|   IBIS model for TI xxx DSP
[IBIS Ver]   5.1
[Disclaimer]   Please be aware that in the absence of a written agreement
|   Texas Instruments(TI) assumes no liability for:
|   (1) The accuracy of the IBIS models provided to your company,
|   however, the IBIS model is compliant to industry standard
|   IQ Level 2a.  Refer to IBIS Quality Section below for
|   for full details.
|   (2) The proper functioning of these Models in your design
|   or for any resulting applications
|   (3) Infringement of patents, copyrights or intellectual
|   property rights resulting from your use of these
|   models.
|   TI provides IBIS Models as a service to our customers and
|   therefore reserves the right to limit distribution of the
|   Models.  The information is subject to change without notice.
[File Name]  dlp8430_v2.ibs
[File Rev]   0.2
|   -Initial version
|   -updated LVCMOS models
[Date]   11Sept2024
[Source]   Texas Instruments Incorporated
[Copyright]   Property of Texas Instruments Incorporated.
|   Unauthorized reproduction and/or distribution is strictly.
|   prohibited.
|   This product is protected under copyright law and trade
|   secret law as an unpublished work.
|   Created 2012,(C) Copyright 1999-2012,
|   Texas Instruments Incorporated., All Rights Reserved.
|   These commodities are under the U.S. Government
|   distribution license control. As such,they are not to be
|   re-exported without the prior approval of the U.S.
|   Department of Commerce.
[Notes]
   This file does not include AMI models for SerDes based links.
   For SerDes simulations use Texas Instruments IBIS AMI models
   Some IV curves contain Non monotonic data points.
|   Revision History
|   GERNERAL COMMENT: All IBIS Quality Notes below reflect latest release
|   and version of IBIS File
|   File passes ibischk6.0 with 0 errors and 139 warnings
|   Component DLP84xx
[Component] DLP84xx
[Manufacturer] Texas Instruments
[Package]
|Variable   Typ   Min   Max
R_pkg   0.139   0.031	0.325
L_pkg   1.052e-9   0.293e-9	2.336e-9
C_pkg   0.364e-12   0.208e-12	0.669e-12
[Package Model]   dlpc84xx_pkg
[Pin]  Signal_name   model_name
A1	VSS   GND
A3	DMD_HS0_WDATA0_P	LVDS
A5	DMD_HS0_WDATA3_P	LVDS
A7	DMD_HS0_WDATA5_P	LVDS
A9	VSS   GND
A11	DMD_HS1_WDATA1_P	LVDS
A13	DMD_HS1_CLK_P   LVDS
A15	DMD_HS1_WDATA6_P	LVDS
A17	DMD_HS2_WDATA0_P	LVDS
A19	DMD_HS2_CLK_P   LVDS
A21	DMD_HS2_WDATA5_P	LVDS
A23	VSS   GND
A25	VSS   GND
B2	DMD_LS0_WDATA_P   LVDS
B4	DMD_HS0_WDATA2_P	LVDS
B6	DMD_HS0_CLK_P   LVDS
B8	DMD_HS0_WDATA7_P	LVDS
B10	DMD_HS1_WDATA0_P	LVDS
B12	DMD_HS1_WDATA3_P	LVDS
B14	DMD_HS1_WDATA4_P	LVDS
B16	VSS   GND
B18	DMD_HS2_WDATA2_P	LVDS
B20	DMD_HS2_WDATA4_P	LVDS
B22	DMD_HS2_WDATA7_P	LVDS
B24	DMD_HS3_WDATA0_P	LVDS
C1	DMD_LS0_WDATA_N	LVDS
C3	DMD_HS0_WDATA0_N	LVDS
C5	DMD_HS0_WDATA3_N	LVDS
C7	DMD_HS0_WDATA5_N	LVDS
C9	VSS   GND
C11	DMD_HS1_WDATA1_N	LVDS
C13	DMD_HS1_CLK_N   LVDS
C15	DMD_HS1_WDATA6_N	LVDS
C17	DMD_HS2_WDATA0_N	LVDS
C19	DMD_HS2_CLK_N   LVDS
C21	DMD_HS2_WDATA5_N	LVDS
C23	VSS   GND
C25	DMD_HS3_WDATA0_N	LVDS
D2	VSS   GND
D4	DMD_HS0_WDATA2_N	LVDS
D6	DMD_HS0_CLK_N   LVDS
D8	DMD_HS0_WDATA7_N	LVDS
D10	DMD_HS1_WDATA0_N	LVDS
D12	DMD_HS1_WDATA3_N	LVDS
D14	DMD_HS1_WDATA4_N	LVDS
D16	VSS   GND
D18	DMD_HS2_WDATA2_N	LVDS
D20	DMD_HS2_WDATA4_N	LVDS
D22	DMD_HS2_WDATA7_N	LVDS
D24	DMD_HS3_WDATA1_P	LVDS
E1	DMD_LS0_CLK_N   LVDS
E3	DMD_LS1_WDATA   LVCMOS18_H
E5	DMD_HS0_WDATA1_N	LVDS
E7	DMD_HS0_WDATA4_N	LVDS
E9	DMD_HS0_WDATA6_N	LVDS
E11	DMD_HS1_WDATA2_N	LVDS
E13	DMD_HS1_WDATA5_N	LVDS
E15	DMD_HS1_WDATA7_N	LVDS
E17	DMD_HS2_WDATA1_N	LVDS
E19	DMD_HS2_WDATA3_N	LVDS
E21	DMD_HS2_WDATA6_N	LVDS
E23	DMD_HS3_WDATA2_N	LVDS
E25	DMD_HS3_WDATA1_N	LVDS
F2	DMD_LS0_CLK_P   LVDS
F4	DMD_HS0_WDATA1_P	LVDS
F6	DMD_HS0_WDATA4_P	LVDS
F8	DMD_HS0_WDATA6_P	LVDS
F10	DMD_HS1_WDATA2_P	LVDS
F12	DMD_HS1_WDATA5_P	LVDS
F14	DMD_HS1_WDATA7_P	LVDS
F16	DMD_HS2_WDATA1_P	LVDS
F18	DMD_HS2_WDATA3_P	LVDS
F20	DMD_HS2_WDATA6_P	LVDS
F22	DMD_HS3_WDATA2_P	LVDS
F24	DMD_HS3_WDATA3_P	LVDS
G1	DMD_LS1_CLK   LVCMOS18_H
G3	DMD_LS2_WDATA   LVCMOS18_H
G5	VSS   GND
G7	VSS   GND
G9	VSS   GND
G11	VSS   GND
G13	ATEST   NC
G15	VSS   GND
G17	VSS   GND
G19	VSS   GND
G21	VSS   GND
G23	DMD_HS3_WDATA4_N	LVDS
G25	DMD_HS3_WDATA3_N	LVDS
H2	DMD_LS2_CLK   LVCMOS18_H
H4	DMD_LS0_RDATA   LVCMOS18_H
H6	VSS   GND
H8	VSS   GND
H10	VSS   GND
H12	VSS   GND
H14	VSS   GND
H16	VSS   GND
H18	VSS   GND
H20	VSS   GND
H22	DMD_HS3_WDATA4_P	LVDS
H24	DMD_HS3_CLK_P   LVDS
J1	DMD_DEN_ARSTZ   LVCMOS18_H
J3	DMD_LS1_RDATA   LVCMOS18_H
J5	VSS   GND
J7	VDDA18_DDI   POWER
J9	VDDA18_DDI   POWER
J11	VDDA18_DDI   POWER
J13	VDDA18_PLLD   POWER
J15	VDDA18_DDI   POWER
J17	VDDA18_DDI   POWER
J19	VDDA18_DDI   POWER
J21	VSS   GND
J23	DMD_HS3_WDATA6_N	LVDS
J25	DMD_HS3_CLK_N   LVDS
K2	VSENSE   NC
K4	DMD_LS3_RDATA   LVCMOS18_H
K6	VSS   GND
K8	VDD_CORE   POWER
K10	VSS   GND
K16	VSS   GND
K18	VDD_CORE   POWER
K20	VSS   GND
K22	DMD_HS3_WDATA6_P	LVDS
K24	DMD_HS3_WDATA5_P	LVDS
L1	PLL_REFCLK_O   NC
L3	IFORCE   NC
L5	VSS   GND
L7	VSS   GND
L9	VDD_CORE   POWER
L11	VSS   GND
L13	VDD_CORE   POWER
L15	VSS   GND
L17	VSS   GND
L21	VPP   NC
L23	DMD_HS3_WDATA7_N	LVDS
L25	DMD_HS3_WDATA5_N	LVDS
M2	VSS   GND
M4	DMD_LS2_RDATA   LVCMOS18_H
M6	VDD_CORE   POWER
M10	VSS   GND
M14	VSS   GND
M18	VSS   GND
M20	VDD_CORE   POWER
M22	DMD_HS3_WDATA7_P	LVDS
M24	TSTPT_7   LVCMOS18_H
N1	PLL_REFCLK_I   NC
N3	GPIO_09   LVCMOS18_H
N5	VSS   GND
N7	VSS   GND
N11	VDDAR_CORE   POWER
N13	VDDAR_CORE   POWER
N15	VDD_CORE   POWER
N17	VDD_CORE   POWER
N21	VDDS18_LVCMOS2   POWER
N23	TSTPT_6   LVCMOS18_H
N25	TSTPT_4   LVCMOS18_H
P2	RESETZ   RESET_H
P4	GPIO_10   LVCMOS18_H
P8	VDDAR_CORE   POWER
P10	VSS   GND
P12	VSS   GND
P14	VSS   GND
P18	VDDAR_CORE   POWER
P20	VSS   GND
P22	TSTPT_5   LVCMOS18_H
P24	TSTPT_3   LVCMOS18_H
R1	GPIO_19   LVCMOS18_H
R3	GPIO_20   LVCMOS18_H
R5	VSS   GND
R9	VDDAR_CORE   POWER
R11	VSS   GND
R15	VSS   GND
R17	VSS   GND
R19	VDDAR_CORE   POWER
R21	VDDS18_LVCMOS2   POWER
R23	TSTPT_2   LVCMOS18_H
R25	TSTPT_1   LVCMOS18_H
T2	GPIO_22   LVCMOS18_H
T4	GPIO_11   LVCMOS18_H
T6	VDD_CORE   POWER
T8	VSS   GND
T10	VSS   GND
T12	VDD_CORE   POWER
T14	VDD_CORE   POWER
T16	VSS   GND
T20	VDD_CORE   POWER
T22	TSTPT_0   LVCMOS18_H
T24	ETM_TRACECTL   LVCMOS18_H
U1	GPIO_21   LVCMOS18_H
U3	GPIO_23   LVCMOS18_H
U5	VDDS18_OSC   POWER
U7	VSS   GND
U11	VSS   GND
U15	VSS   GND
U17	VSS   GND
U19	VDD_CORE   POWER
U21	VDDS18_LVCMOS2   POWER
U23	JTAGTMS1   LVCMOS18_H
U25	ETM_TRACECLK   LVCMOS18_H
V2	GPIO_25   LVCMOS18_H
V4	GPIO_12   LVCMOS18_H
V6	VSS   GND
V8	VDD_CORE   POWER
V10	VDD_CORE   POWER
V12	VSS   GND
V14	VSS   GND
V20	VSS   GND
V22	JTAGTDO1   LVCMOS18_H
V24	JTAGTCK   LVCMOS18_H
W1	GPIO_24   LVCMOS18_H
W3	GPIO_26   LVCMOS18_H
W5	VDDS18_LVCMOS1   POWER
W7	VSS   GND
W13	VSS   GND
W15	VDDAR_CORE   POWER
W17	VDDAR_CORE   POWER
W19	VSS   GND
W21	VDDS18_LVCMOS2   POWER
W23	JTAGTDO2   LVCMOS18_H
W25	JTAGTMS2   LVCMOS18_H
Y2	GPIO_29   LVCMOS18_H
Y4	GPIO_28   LVCMOS18_H
Y6	VDD_CORE   POWER
Y8	VSS   GND
Y10	VSS   GND
Y12	VSS   GND
Y14	VSS   GND
Y18	VSS   GND
Y20	VDD_CORE   POWER
Y22	HWTEST_EN   LVCMOS18_H
Y24	JTAGTDI   LVCMOS18_H
AA1	GPIO_27   LVCMOS18_H
AA3	GPIO_30   LVCMOS18_H
AA5	VDDS18_LVCMOS1   POWER
AA7	VSS   GND
AA9	VSS   GND
AA13	VDD_CORE   POWER
AA15	VDD_CORE   POWER
AA17	VSS   GND
AA19	VSS   GND
AA21	VDD_CORE   POWER
AA23	GPTP0   LVCMOS18_H
AA25	JTAGTRSTZ   LVCMOS18_H
AB2	GPIO_33   LVCMOS18_H
AB4	GPIO_31   LVCMOS18_H
AB6	VSS   GND
AB8	VSS   GND
AB10	VDDAR_CORE   POWER
AB12	VDDAR_CORE   POWER
AB14	VSS   GND
AB16	VDD_CORE   POWER
AB18	VSS   GND
AB20	VSS   GND
AB22	GPTP1   LVCMOS18_H
AB24	OCLKA   LVCMOS18_H
AC1	GPIO_32   LVCMOS18_H
AC3	GPIO_34   LVCMOS18_H
AC5	VSS   GND
AC9	VSS   GND
AC11	VSS   GND
AC13	VDD_CORE   POWER
AC15	VSS   GND
AC17	VSS   GND
AC21	VDDSHV_FLSH   POWER
AC23	GPIO_14   LVCMOS18_H
AC25	GPTP2   LVCMOS18_H
AD2	GPIO_37   LVCMOS18_H
AD4	GPIO_35   LVCMOS18_H
AD6	VDD_CORE   POWER
AD8	VDD_CORE   POWER
AD12	VSS   GND
AD14	VSS   GND
AD16	VSS   GND
AD18	VDD_CORE   POWER
AD20	VDD_CORE   POWER
AD22	CAP_VDDS_FLSH   POWER
AD24	GPIO_13   LVCMOS18_H
AE1	GPIO_36   LVCMOS18_H
AE3	GPIO_38   LVCMOS18_H
AE5	VDDS18_LVCMOS1   POWER
AE9	VDD_CORE   POWER
AE11	VDD_CORE   POWER
AE13	VSS   GND
AE17	VSS   GND
AE21	VDDSHV_FLSH   POWER
AE23	GPIO_16   LVCMOS18_H
AE25	GPIO_15   LVCMOS18_H
AF2	GPIO_41   LVCMOS18_H
AF4	GPIO_40   LVCMOS18_H
AF6	VSS   GND
AF8	VSS   GND
AF12	VSS   GND
AF14	VDD_CORE   POWER
AF16	VDD_CORE   POWER
AF18	VSS   GND
AF20	VDD_CORE   POWER
AF22	GPIO_18   LVCMOS18_H
AF24	GPIO_17   LVCMOS18_H
AG1	GPIO_39   LVCMOS18_H
AG3	GPIO_43   LVCMOS18_H
AG5	VDDS18_LVCMOS1   POWER
AG7	VDD_CORE   POWER
AG9	VSS   GND
AG11	VSS   GND
AG13	VSS   GND
AG17	VSS   GND
AG19	VSS   GND
AG21	VDDSHV_INTF   POWER
AG23	FLSH_CSZ   SDIO_H
AG25	FLSH_CLK   SDIO_H
AH2	GPIO_44   LVCMOS18_H
AH4	ATB_0_H   NC
AH6	VDD_CORE   POWER
AH10	VSS   GND
AH14	VSS   GND
AH16	VSS   GND
AH20	VSS   GND
AH22	FLSH_DATA0   SDIO_H
AH24	FLSH_DATA1   SDIO_H
AJ1	GPIO_42   LVCMOS18_H
AJ3	GPIO_45   LVCMOS18_H
AJ5	ATB_1_H   NC
AJ9	VDDAR_CORE   POWER
AJ11	VDD_CORE   POWER
AJ13	VDDAR_CORE   POWER
AJ15	VDDAR_CORE   POWER
AJ17	VDDAR_CORE   POWER
AJ19	VDDAR_CORE   POWER
AJ21	CAP_VDDS_INTF   POWER
AJ23	FLSH_DATA3   SDIO_H
AJ25	FLSH_DATA2   SDIO_H
AK2	GPIO_48   LVCMOS18_H
AK4	GPIO_47   LVCMOS18_H
AK6	VSS   GND
AK8	VDDAR_CORE   POWER
AK16	VSS   GND
AK20	VSS   GND
AK22	HOST_IRQ   LVCMOS1833_H
AK24	IIC0_SDA   IIC_H
AL1	GPIO_46   LVCMOS18_H
AL3	GPIO_50   LVCMOS18_H
AL5	VDDS18_LVCMOS1   POWER
AL7	VSS   GND
AL9	VDD_CORE   POWER
AL11	VDDA18_PLLM   POWER
AL13	VDD_CORE   POWER
AL15	VSS   GND
AL17	VDD_CORE   POWER
AL19	VDD_CORE   POWER
AL21	VDDSHV_INTF   POWER
AL23	GPIO_07   LVCMOS1833_H
AL25	IIC0_SCL   IIC_H
AM2	GPIO_51   LVCMOS18_H
AM4	P1_LOCKN   LVCMOS18_H
AM6	VDDA_CORE_USB   POWER
AM8	VSS   GND
AM10	VDDA_CORE_VX1   POWER
AM12	VDDA18_VX1   POWER
AM14	VDDA_CORE_VX1   POWER
AM16	VDDA_CORE_FPD   POWER
AM18	VDDA_CORE_FPD   POWER
AM20	VDDA_CORE_FPD   POWER
AM22	SSP0_CSZ_0   LVCMOS1833_H
AM24	GPIO_08   LVCMOS1833_H
AN1	GPIO_49   LVCMOS18_H
AN3	P1_HTPDN   LVCMOS18_H
AN5	VSS   GND
AN7	VDDA18_USB   POWER
AN9	VSS   GND
AN15	VDDA18_FPD   POWER
AN21	VSS   GND
AN23	SSP0_DI   LVCMOS1833_H
AN25	SSP0_CLK   LVCMOS1833_H
AP2	PROJ_ON   LVCMOS18_H
AP4	USB_VBUS   NC
AP6	VDDA33_USB   POWER
AP8	VDDA18_DSI   POWER
AP10	VDDA18_VX1   POWER
AP12	VSS   GND
AP14	VDDA18_VX1   POWER
AP16	VDDA18_FPD   POWER
AP18	VDDA18_FPD   POWER
AP20	VSS   GND
AP22	GPIO_06   LVCMOS1833_H
AP24	SSP0_DO   LVCMOS1833_H
AR1	PARKZ   LVCMOS18_H
AR3	USB_TXRTUNE   NC
AR5	VSS   GND
AR7	VDDA_CORE_DSI   POWER
AR9	VSS   GND
AR11	VSS   GND
AR13	VSS   GND
AR15	VSS   GND
AR17	VSS   GND
AR19	VDDA18_FPD   POWER
AR21	VSS   GND
AR23	GPIO_05   LVCMOS1833_H
AR25	GPIO_00   LVCMOS1833_H
AT2	USB_ID   NC
AT4	VSS   GND
AT6	VSS   GND
AT8	VSS   GND
AT10	VSS   GND
AT12	VSS   GND
AT14	VSS   GND
AT16	P2A_LVDS_RPI   NC
AT18	VSS   GND
AT20	P2B_LVDS_RPI   NC
AT22	VSS   GND
AT24	GPIO_03   LVCMOS1833_H
AU1	USB_DAT_P   NC
AU3	VSS   GND
AU5	P3_DSI_D2_N   NC
AU7	VSS   GND
AU9	P1_VX1_D0_N   VBO
AU11	P1_RREF   NC
AU13	P1_VX1_D5_N   VBO
AU15	P2A_LVDS_D2_N   FPD
AU17	P2A_LVDS_D4_N   FPD
AU19	P2B_LVDS_D1_N   FPD
AU21	P2B_LVDS_D2_N   FPD
AU23	VSS   GND
AU25	GPIO_01   LVCMOS1833_H
AV2	VSS   GND
AV4	P3_DSI_D2_P   NC
AV6	P3_DSI_RCALIB   NC
AV8	P1_VX1_D0_P   VBO
AV10	VSS   GND
AV12	P1_VX1_D5_P   NC
AV14	VSS   GND
AV16	P2A_LVDS_D2_P   FPD
AV18	P2A_LVDS_D4_P   FPD
AV20	P2B_LVDS_D1_P   FPD
AV22	P2B_LVDS_D2_P   FPD
AV24	GPIO_04   LVCMOS1833_H
AW1	USB_DAT_N   NC
AW3	P3_DSI_D3_N   NC
AW5	P3_DSI_D0_N   NC
AW7	VSS   GND
AW9	P1_VX1_D2_N   VBO
AW11	P1_VX1_D4_N   VBO
AW13	P1_VX1_D7_N   VBO
AW15	P2A_LVDS_D0_N   FPD
AW17	P2A_LVDS_C_N   FPD
AW19	VSS   GND
AW21	P2B_LVDS_C_N   FPD
AW23	P2B_LVDS_D4_N   FPD
AW25	GPIO_02   LVCMOS1833_H
AY2	VSS   GND
AY4	P3_DSI_D1_N   NC
AY6	P3_DSI_C_N   NC
AY8	P1_VX1_D1_N   VBO
AY10	P1_VX1_D3_N   VBO
AY12	P1_VX1_D6_N   VBO
AY14	VSS   GND
AY16	P2A_LVDS_D1_N   FPD
AY18	P2A_LVDS_D3_N   FPD
AY20	P2B_LVDS_D0_N   FPD
AY22	P2B_LVDS_D3_N   FPD
AY24	VSS   GND
BA1	VSS   GND
BA3	P3_DSI_D3_P   NC
BA5	P3_DSI_D0_P   NC
BA7	VSS   GND
BA9	P1_VX1_D2_P   VBO
BA11	P1_VX1_D4_P   VBO
BA13	P1_VX1_D7_P   VBO
BA15	P2A_LVDS_D0_P   FPD
BA17	P2A_LVDS_C_P   FPD
BA19	VSS   GND
BA21	P2B_LVDS_C_P   FPD
BA23	P2B_LVDS_D4_P   FPD
BA25	VSS   GND
BB2	VSS   GND
BB4	P3_DSI_D1_P   NC
BB6	P3_DSI_C_P   NC
BB8	P1_VX1_D1_P   VBO
BB10	P1_VX1_D3_P   VBO
BB12	P1_VX1_D6_P   VBO
BB14	VSS   GND
BB16	P2A_LVDS_D1_P   FPD
BB18	P2A_LVDS_D3_P   FPD
BB20	P2B_LVDS_D0_P   FPD
BB22	P2B_LVDS_D3_P   FPD
BB24	VSS   GND
|********************  DIFF PIN  *******************************
[Diff_pin]   inv_pin vdiff tdelay_typ   tdelay_min  tdelay_max
B6   D6   NA NA NA NA	||	DMD_HS0_CLK_P && DMD_HS0_CLK_N
A3   C3   NA NA NA NA	||	DMD_HS0_WDATA0_P && DMD_HS0_WDATA0_N
F4   E5   NA NA NA NA	||	DMD_HS0_WDATA1_P && DMD_HS0_WDATA1_N
B4   D4   NA NA NA NA	||	DMD_HS0_WDATA2_P && DMD_HS0_WDATA2_N
A5   C5   NA NA NA NA	||	DMD_HS0_WDATA3_P && DMD_HS0_WDATA3_N
F6   E7   NA NA NA NA	||	DMD_HS0_WDATA4_P && DMD_HS0_WDATA4_N
A7   C7   NA NA NA NA	||	DMD_HS0_WDATA5_P && DMD_HS0_WDATA5_N
F8   E9   NA NA NA NA	||	DMD_HS0_WDATA6_P && DMD_HS0_WDATA6_N
B8   D8   NA NA NA NA	||	DMD_HS0_WDATA7_P && DMD_HS0_WDATA7_N
A13   C13   NA NA NA NA	||	DMD_HS1_CLK_P && DMD_HS1_CLK_N
B10   D10   NA NA NA NA	||	DMD_HS1_WDATA0_P && DMD_HS1_WDATA0_N
A11   C11   NA NA NA NA	||	DMD_HS1_WDATA1_P && DMD_HS1_WDATA1_N
F10   E11   NA NA NA NA	||	DMD_HS1_WDATA2_P && DMD_HS1_WDATA2_N
B12   D12   NA NA NA NA	||	DMD_HS1_WDATA3_P && DMD_HS1_WDATA3_N
B14   D14   NA NA NA NA	||	DMD_HS1_WDATA4_P && DMD_HS1_WDATA4_N
F12   E13   NA NA NA NA	||	DMD_HS1_WDATA5_P && DMD_HS1_WDATA5_N
A15   C15   NA NA NA NA	||	DMD_HS1_WDATA6_P && DMD_HS1_WDATA6_N
F14   E15   NA NA NA NA	||	DMD_HS1_WDATA7_P && DMD_HS1_WDATA7_N
A19   C19   NA NA NA NA	||	DMD_HS2_CLK_P && DMD_HS2_CLK_N
A17   C17   NA NA NA NA	||	DMD_HS2_WDATA0_P && DMD_HS2_WDATA0_N
F16   E17   NA NA NA NA	||	DMD_HS2_WDATA1_P && DMD_HS2_WDATA1_N
B18   D18   NA NA NA NA	||	DMD_HS2_WDATA2_P && DMD_HS2_WDATA2_N
F18   E19   NA NA NA NA	||	DMD_HS2_WDATA3_P && DMD_HS2_WDATA3_N
B20   D20   NA NA NA NA	||	DMD_HS2_WDATA4_P && DMD_HS2_WDATA4_N
A21   C21   NA NA NA NA	||	DMD_HS2_WDATA5_P && DMD_HS2_WDATA5_N
F20   E21   NA NA NA NA	||	DMD_HS2_WDATA6_P && DMD_HS2_WDATA6_N
B22   D22   NA NA NA NA	||	DMD_HS2_WDATA7_P && DMD_HS2_WDATA7_N
H24   J25   NA NA NA NA	||	DMD_HS3_CLK_P && DMD_HS3_CLK_N
B24   C25   NA NA NA NA	||	DMD_HS3_WDATA0_P && DMD_HS3_WDATA0_N
D24   E25   NA NA NA NA	||	DMD_HS3_WDATA1_P && DMD_HS3_WDATA1_N
F22   E23   NA NA NA NA	||	DMD_HS3_WDATA2_P && DMD_HS3_WDATA2_N
F24   G25   NA NA NA NA	||	DMD_HS3_WDATA3_P && DMD_HS3_WDATA3_N
H22   G23   NA NA NA NA	||	DMD_HS3_WDATA4_P && DMD_HS3_WDATA4_N
K24   L25   NA NA NA NA	||	DMD_HS3_WDATA5_P && DMD_HS3_WDATA5_N
K22   J23   NA NA NA NA	||	DMD_HS3_WDATA6_P && DMD_HS3_WDATA6_N
M22   L23   NA NA NA NA	||	DMD_HS3_WDATA7_P && DMD_HS3_WDATA7_N
F2   E1   NA NA NA NA	||	DMD_LS0_CLK_P && DMD_LS0_CLK_N
B2   C1   NA NA NA NA	||	DMD_LS0_WDATA_P && DMD_LS0_WDATA_N
AV8   AU9   NA NA NA NA	||	P1_VX1_D0_P && P1_VX1_D0_N
BB8   AY8   NA NA NA NA	||	P1_VX1_D1_P && P1_VX1_D1_N
BA9   AW9   NA NA NA NA	||	P1_VX1_D2_P && P1_VX1_D2_N
BB10   AY10   NA NA NA NA	||	P1_VX1_D3_P && P1_VX1_D3_N
BA11   AW11   NA NA NA NA	||	P1_VX1_D4_P && P1_VX1_D4_N
AV12   AU13   NA NA NA NA	||	P1_VX1_D5_P && P1_VX1_D5_N
BB12   AY12   NA NA NA NA	||	P1_VX1_D6_P && P1_VX1_D6_N
BA13   AW13   NA NA NA NA	||	P1_VX1_D7_P && P1_VX1_D7_N
BA17   AW17   NA NA NA NA	||	P2A_LVDS_C_P && P2A_LVDS_C_N
BA15   AW15   NA NA NA NA	||	P2A_LVDS_D0_P && P2A_LVDS_D0_N
BB16   AY16   NA NA NA NA	||	P2A_LVDS_D1_P && P2A_LVDS_D1_N
AV16   AU15   NA NA NA NA	||	P2A_LVDS_D2_P && P2A_LVDS_D2_N
BB18   AY18   NA NA NA NA	||	P2A_LVDS_D3_P && P2A_LVDS_D3_N
AV18   AU17   NA NA NA NA	||	P2A_LVDS_D4_P && P2A_LVDS_D4_N
BA21   AW21   NA NA NA NA	||	P2B_LVDS_C_P && P2B_LVDS_C_N
BB20   AY20   NA NA NA NA	||	P2B_LVDS_D0_P && P2B_LVDS_D0_N
AV20   AU19   NA NA NA NA	||	P2B_LVDS_D1_P && P2B_LVDS_D1_N
AV22   AU21   NA NA NA NA	||	P2B_LVDS_D2_P && P2B_LVDS_D2_N
BB22   AY22   NA NA NA NA	||	P2B_LVDS_D3_P && P2B_LVDS_D3_N
BA23   AW23   NA NA NA NA	||	P2B_LVDS_D4_P && P2B_LVDS_D4_N
|******************** LVDS ***********************************
[Model Selector] LVDS
lvds_tx_01   LVDS TX Driver Permumentation 01
lvds_tx_02   LVDS TX Driver Permumentation 02
lvds_tx_03   LVDS TX Driver Permumentation 03
lvds_tx_04   LVDS TX Driver Permumentation 04
lvds_tx_05   LVDS TX Driver Permumentation 05
lvds_tx_06   LVDS TX Driver Permumentation 06
lvds_tx_07   LVDS TX Driver Permumentation 07
lvds_tx_08   LVDS TX Driver Permumentation 08
lvds_tx_09   LVDS TX Driver Permumentation 09
lvds_tx_10   LVDS TX Driver Permumentation 10
lvds_tx_11   LVDS TX Driver Permumentation 11
lvds_tx_12   LVDS TX Driver Permumentation 12
lvds_tx_13   LVDS TX Driver Permumentation 13
lvds_tx_14   LVDS TX Driver Permumentation 14
lvds_tx_15   LVDS TX Driver Permumentation 15
lvds_tx_16   LVDS TX Driver Permumentation 16
lvds_tx_17   LVDS TX Driver Permumentation 17
lvds_tx_18   LVDS TX Driver Permumentation 18
lvds_tx_19   LVDS TX Driver Permumentation 19
lvds_tx_20   LVDS TX Driver Permumentation 20
lvds_tx_21   LVDS TX Driver Permumentation 21
lvds_tx_22   LVDS TX Driver Permumentation 22
lvds_tx_23   LVDS TX Driver Permumentation 23
lvds_tx_24   LVDS TX Driver Permumentation 24
|****************** SDIO **************************************
[Model Selector] SDIO_H
sdio1_r33_1p8_h PRWDWUWSWEWCDGSDIO_H@_R33_1p8_comment
sdio1_r33_3p3_h PRWDWUWSWEWCDGSDIO_H@_R33_3p3_comment
sdio1_r40_1p8_h PRWDWUWSWEWCDGSDIO_H@_R40_1p8_comment
sdio1_r40_3p3_h PRWDWUWSWEWCDGSDIO_H@_R40_3p3_comment
sdio1_r50_1p8_h PRWDWUWSWEWCDGSDIO_H@_R50_1p8_comment
sdio1_r50_3p3_h PRWDWUWSWEWCDGSDIO_H@_R50_3p3_comment
sdio1_r66_1p8_h PRWDWUWSWEWCDGSDIO_H@_R66_1p8_comment
sdio1_r66_3p3_h PRWDWUWSWEWCDGSDIO_H@_R66_3p3_comment
sdio1_utr33_1p8_h PRWDWUWSWEWCDGSDIO_H@_UT_R33_1p8_comment
sdio1_utr33_3p3_h PRWDWUWSWEWCDGSDIO_H@_UT_R33_3p3_comment
sdio1_utr40_1p8_h PRWDWUWSWEWCDGSDIO_H@_UT_R40_1p8_comment
sdio1_utr40_3p3_h PRWDWUWSWEWCDGSDIO_H@_UT_R40_3p3_comment
sdio1_utr50_1p8_h PRWDWUWSWEWCDGSDIO_H@_UT_R50_1p8_comment
sdio1_utr50_3p3_h PRWDWUWSWEWCDGSDIO_H@_UT_R50_3p3_comment
sdio1_utr66_1p8_h PRWDWUWSWEWCDGSDIO_H@_UT_R66_1p8_comment
sdio1_utr66_3p3_h PRWDWUWSWEWCDGSDIO_H@_UT_R66_3p3_comment
|********************I2C************************************
[Model Selector] IIC_V
IIC18_1_0_V PRBOPDDGZIIC_V@HSMODE_HSMCSE=0_0_comment 1.8V
IIC18_1_1_V PRBOPDDGZIIC_V@HSMODE_HSMCSE=0_1_comment 1.8V
IIC18_1_2_V PRBOPDDGZIIC_V@HSMODE_HSMCSE=1_0_comment 1.8V
IIC18_1_3_V PRBOPDDGZIIC_V@HSMODE_HSMCSE=1_1_comment 1.8V
IIC33_1_0_V PRBOPDDGZIIC_V@HSMODE_HSMCSE=0_0_comment
IIC33_1_1_V PRBOPDDGZIIC_V@HSMODE_HSMCSE=0_1_comment
IIC33_1_2_V PRBOPDDGZIIC_V@HSMODE_HSMCSE=1_0_comment
IIC33_1_3_V PRBOPDDGZIIC_V@HSMODE_HSMCSE=1_1_comment
[Model Selector] IIC_H
Cell18_0_0_H PRBOPDDGZIIC_H@HSMODE_HSMCSE=0_0_comment 1.8V
Cell18_0_1_H PRBOPDDGZIIC_H@HSMODE_HSMCSE=0_1_comment 1.8V
Cell18_0_2_H PRBOPDDGZIIC_H@HSMODE_HSMCSE=1_0_comment 1.8V
Cell18_0_3_H PRBOPDDGZIIC_H@HSMODE_HSMCSE=1_1_comment 1.8V
Cell33_0_0_H PRBOPDDGZIIC_H@HSMODE_HSMCSE=0_0_comment
Cell33_0_1_H PRBOPDDGZIIC_H@HSMODE_HSMCSE=0_1_comment
Cell33_0_2_H PRBOPDDGZIIC_H@HSMODE_HSMCSE=1_0_comment
Cell33_0_3_H PRBOPDDGZIIC_H@HSMODE_HSMCSE=1_1_comment
|***************** RESET *********************************************
[Model Selector] RESET_H
reset18_0_0 PDIDGZRESET_H
| **************** LVCMOS18 ******************************************
[Model Selector] LVCMOS18_H
|Cell1_0 PRWDWUWHWSWDGZ_H@DS0_DS1_DS2_DS3_SL_PE_PS_SPU=0_0_0_0_0_0_0_0_comment
|Cell1_1 PRWDWUWHWSWDGZ_H@DS0_DS1_DS2_DS3_SL_PE_PS_SPU=0_0_0_0_1_0_0_0_comment
|Cell1_2 PRWDWUWHWSWDGZ_H@DS0_DS1_DS2_DS3_SL_PE_PS_SPU=0_0_0_1_0_0_0_0_comment
|Cell1_3 PRWDWUWHWSWDGZ_H@DS0_DS1_DS2_DS3_SL_PE_PS_SPU=0_0_0_1_1_0_0_0_comment
|Cell1_4 PRWDWUWHWSWDGZ_H@DS0_DS1_DS2_DS3_SL_PE_PS_SPU=0_0_1_0_0_0_0_0_comment
|Cell1_5 PRWDWUWHWSWDGZ_H@DS0_DS1_DS2_DS3_SL_PE_PS_SPU=0_0_1_0_1_0_0_0_comment
|Cell1_6 PRWDWUWHWSWDGZ_H@DS0_DS1_DS2_DS3_SL_PE_PS_SPU=0_0_1_1_0_0_0_0_comment
|Cell1_7 PRWDWUWHWSWDGZ_H@DS0_DS1_DS2_DS3_SL_PE_PS_SPU=0_0_1_1_1_0_0_0_comment
|Cell1_8 PRWDWUWHWSWDGZ_H@DS0_DS1_DS2_DS3_SL_PE_PS_SPU=0_1_0_0_0_0_0_0_comment
|Cell1_9 PRWDWUWHWSWDGZ_H@DS0_DS1_DS2_DS3_SL_PE_PS_SPU=0_1_0_0_1_0_0_0_comment
|Cell1_10 PRWDWUWHWSWDGZ_H@DS0_DS1_DS2_DS3_SL_PE_PS_SPU=0_1_0_1_0_0_0_0_comment
|Cell1_11 PRWDWUWHWSWDGZ_H@DS0_DS1_DS2_DS3_SL_PE_PS_SPU=0_1_0_1_1_0_0_0_comment
|Cell1_12 PRWDWUWHWSWDGZ_H@DS0_DS1_DS2_DS3_SL_PE_PS_SPU=0_1_1_0_0_0_0_0_comment
|Cell1_13 PRWDWUWHWSWDGZ_H@DS0_DS1_DS2_DS3_SL_PE_PS_SPU=0_1_1_0_1_0_0_0_comment
|Cell1_14 PRWDWUWHWSWDGZ_H@DS0_DS1_DS2_DS3_SL_PE_PS_SPU=0_1_1_1_0_0_0_0_comment
|Cell1_15 PRWDWUWHWSWDGZ_H@DS0_DS1_DS2_DS3_SL_PE_PS_SPU=0_1_1_1_1_0_0_0_comment
|Cell1_16 PRWDWUWHWSWDGZ_H@DS0_DS1_DS2_DS3_SL_PE_PS_SPU=1_0_0_0_0_0_0_0_comment
|Cell1_17 PRWDWUWHWSWDGZ_H@DS0_DS1_DS2_DS3_SL_PE_PS_SPU=1_0_0_0_1_0_0_0_comment
|Cell1_18 PRWDWUWHWSWDGZ_H@DS0_DS1_DS2_DS3_SL_PE_PS_SPU=1_0_0_1_0_0_0_0_comment
|Cell1_19 PRWDWUWHWSWDGZ_H@DS0_DS1_DS2_DS3_SL_PE_PS_SPU=1_0_0_1_1_0_0_0_comment
Cell1_20 PRWDWUWHWSWDGZ_H@DS0_DS1_DS2_DS3_SL_PE_PS_SPU=1_0_1_0_0_0_0_0_comment
Cell1_21 PRWDWUWHWSWDGZ_H@DS0_DS1_DS2_DS3_SL_PE_PS_SPU=1_0_1_0_1_0_0_0_comment
|Cell1_22 PRWDWUWHWSWDGZ_H@DS0_DS1_DS2_DS3_SL_PE_PS_SPU=1_0_1_1_0_0_0_0_comment
|Cell1_23 PRWDWUWHWSWDGZ_H@DS0_DS1_DS2_DS3_SL_PE_PS_SPU=1_0_1_1_1_0_0_0_comment
|Cell1_24 PRWDWUWHWSWDGZ_H@DS0_DS1_DS2_DS3_SL_PE_PS_SPU=1_1_0_0_0_0_0_0_comment
|Cell1_25 PRWDWUWHWSWDGZ_H@DS0_DS1_DS2_DS3_SL_PE_PS_SPU=1_1_0_0_1_0_0_0_comment
|Cell1_26 PRWDWUWHWSWDGZ_H@DS0_DS1_DS2_DS3_SL_PE_PS_SPU=1_1_0_1_0_0_0_0_comment
|Cell1_27 PRWDWUWHWSWDGZ_H@DS0_DS1_DS2_DS3_SL_PE_PS_SPU=1_1_0_1_1_0_0_0_comment
|Cell1_28 PRWDWUWHWSWDGZ_H@DS0_DS1_DS2_DS3_SL_PE_PS_SPU=1_1_1_0_0_0_0_0_comment
|Cell1_29 PRWDWUWHWSWDGZ_H@DS0_DS1_DS2_DS3_SL_PE_PS_SPU=1_1_1_0_1_0_0_0_comment
|Cell1_30 PRWDWUWHWSWDGZ_H@DS0_DS1_DS2_DS3_SL_PE_PS_SPU=1_1_1_1_0_0_0_0_comment
|Cell1_31 PRWDWUWHWSWDGZ_H@DS0_DS1_DS2_DS3_SL_PE_PS_SPU=1_1_1_1_1_0_0_0_comment
[Model Selector] LVCMOS1833_H
lvcmos1_nom_1p8_h PRWDWUWSWEWCDGLVCMOS_V@DS3_DS2_DS1_DS0=1_1_0_0_comment
lvcmos1_nom_3p3_h PRWDWUWSWEWCDGLVCMOS_V@DS3_DS2_DS1_DS0=1_1_0_0_comment
|lvcmos1_nom_1p8_h PRWDWUWSWEWCDGLVCMOS_H@_Nom_1p8_comment
|lvcmos1_nom_3p3_h PRWDWUWSWEWCDGLVCMOS_H@_Nom_3p3_comment
|vcmos1_slow_1p8_h PRWDWUWSWEWCDGLVCMOS_H@_Slow_1p8_comment
|vcmos1_slow_3p3_h PRWDWUWSWEWCDGLVCMOS_H@_Slow_3p3_comment
|vcmos1_fast_1p8_h PRWDWUWSWEWCDGLVCMOS_H@_Fast_1p8_comment
|vcmos1_fast_3p3_h PRWDWUWSWEWCDGLVCMOS_H@_Fast_3p3_comment
|vcmos1_utnom_1p8_h PRWDWUWSWEWCDGLVCMOS_H@_UT_Nom_1p8_comment
|vcmos1_utnom_3p3_h PRWDWUWSWEWCDGLVCMOS_H@_UT_Nom_3p3_comment
|vcmos1_utslow_1p8_h PRWDWUWSWEWCDGLVCMOS_H@_UT_Slow_1p8_comment
|vcmos1_utslow_3p3_h PRWDWUWSWEWCDGLVCMOS_H@_UT_Slow_3p3_comment
|vcmos1_utfast_1p8_h PRWDWUWSWEWCDGLVCMOS_H@_UT_Fast_1p8_comment
|vcmos1_utfast_3p3_h PRWDWUWSWEWCDGLVCMOS_H@_UT_Fast_3p3_comment
[Model Selector] LVCMOS1833_V
lvcmos0_nom_1p8_v PRWDWUWSWEWCDGLVCMOS_H@DS3_DS2_DS1_DS0=1_1_0_0_comment
lvcmos0_nom_3p3_v PRWDWUWSWEWCDGLVCMOS_H@DS3_DS2_DS1_DS0=1_1_0_0_comment
|lvcmos0_nom_1p8_v PRWDWUWSWEWCDGLVCMOS_V@_Nom_1p8_comment
|lvcmos0_nom_3p3_v PRWDWUWSWEWCDGLVCMOS_V@_Nom_3p3_comment
|vcmos0_slow_1p8_v PRWDWUWSWEWCDGLVCMOS_V@_Slow_1p8_comment
|vcmos0_slow_3p3_v PRWDWUWSWEWCDGLVCMOS_V@_Slow_3p3_comment
|vcmos0_fast_1p8_v PRWDWUWSWEWCDGLVCMOS_V@_Fast_1p8_comment
|vcmos0_fast_3p3_v PRWDWUWSWEWCDGLVCMOS_V@_Fast_3p3_comment
|vcmos0_utnom_1p8_v PRWDWUWSWEWCDGLVCMOS_V@_UT_Nom_1p8_comment
|vcmos0_utnom_3p3_v PRWDWUWSWEWCDGLVCMOS_V@_UT_Nom_3p3_comment
|vcmos0_utslow_1p8_v PRWDWUWSWEWCDGLVCMOS_V@_UT_Slow_1p8_comment
|vcmos0_utslow_3p3_v PRWDWUWSWEWCDGLVCMOS_V@_UT_Slow_3p3_comment
|vcmos0_utfast_1p8_v PRWDWUWSWEWCDGLVCMOS_V@_UT_Fast_1p8_comment
|vcmos0_utfast_3p3_v PRWDWUWSWEWCDGLVCMOS_V@_UT_Fast_3p3_comment
| ********************** LVDS *********************************************
| ********************** FPD **********************************************
[Model Selector] FPD
FPD_RX_P   FPD RX P
FPD_RX_N   FPD RX N
| ********************** VBO **********************************************
[Model Selector] VBO
VBO_RX_P   VBO RX P
VBO_RX_N   VBO RX N
|**************** Package Model **********************************
[Define Package Model]   dlpc84xx_pkg
[Manufacturer]   name 1
[OEM]   name 2
[Description]   265-pin Package
|[Number of Sections]   1
[Number of Pins]   265
[Pin Numbers]
|[Pin Name]  Net Number   Net Name   Net's All Pins
AD22   | 1   CAP_VDDS_FLSH   AD22
AJ21   | 2   CAP_VDDS_INTF   AJ21
J7   | 3   VDDA18_DDI   J7
   |J9
   |J11
   |J15
   |J17
   |J19
AP8   | 4   VDDA18_DSI   AP8
J13   | 5   VDDA18_PLLD   J13
AL11   | 6   VDDA18_PLLM   AL11
AN7   | 7   VDDA18_USB   AN7
AM12   | 8   VDDA18_VX1   AM12
   |AP10
   |AP14
AP6   | 9   VDDA33_USB   AP6
AB10   | 10   VDDAR_CORE   AB10
   |AB12
   |AJ9
   |AJ13
   |AJ15
   |AJ17
   |AJ19
   |AK8
   |N11
   |N13
   |P8
   |P18
   |R9
   |R19
   |W15
   |W17
AR7   | 11   VDDA_CORE_DSI   AR7
AM6   | 12   VDDA_CORE_USB   AM6
AM10   | 13   VDDA_CORE_VX1   AM10
   |AM14
AA5   | 14   VDDS18_LVCMOS1   AA5
   |AE5
   |AG5
   |AL5
   |W5
N21   | 15   VDDS18_LVCMOS2   N21
   |R21
   |U21
   |W21
U5   | 16   VDDS18_OSC   U5
AC21   | 17   VDDSHV_FLSH   AC21
   |AE21
AG21   | 18   VDDSHV_INTF   AG21
   |AL21
AA13   | 19   VDD_CORE   AA13
   |AA15
   |AA21
   |AB16
   |AC13
   |AD6
   |AD8
   |AD18
   |AD20
   |AE9
   |AE11
   |AF14
   |AF16
   |AF20
   |AG7
   |AH6
   |AJ11
   |AL9
   |AL13
   |AL17
   |AL19
   |K8
   |K18
   |L9
   |L13
   |M6
   |M20
   |N15
   |N17
   |T6
   |T12
   |T14
   |T20
   |U19
   |V8
   |V10
   |Y6
   |Y20
L21   | 20   VPP   L21
AH4   | 21   ATB_0_H   AH4
AJ5   | 22   ATB_1_H   AJ5
G13   | 23   ATEST   G13
J1   | 24   DMD_DEN_ARSTZ   J1
D6   | 25   DMD_HS0_CLK_N   D6
B6   | 26   DMD_HS0_CLK_P   B6
C3   | 27   DMD_HS0_WDATA0_N   C3
A3   | 28   DMD_HS0_WDATA0_P   A3
E5   | 29   DMD_HS0_WDATA1_N   E5
F4   | 30   DMD_HS0_WDATA1_P   F4
D4   | 31   DMD_HS0_WDATA2_N   D4
B4   | 32   DMD_HS0_WDATA2_P   B4
C5   | 33   DMD_HS0_WDATA3_N   C5
A5   | 34   DMD_HS0_WDATA3_P   A5
E7   | 35   DMD_HS0_WDATA4_N   E7
F6   | 36   DMD_HS0_WDATA4_P   F6
C7   | 37   DMD_HS0_WDATA5_N   C7
A7   | 38   DMD_HS0_WDATA5_P   A7
E9   | 39   DMD_HS0_WDATA6_N   E9
F8   | 40   DMD_HS0_WDATA6_P   F8
D8   | 41   DMD_HS0_WDATA7_N   D8
B8   | 42   DMD_HS0_WDATA7_P   B8
C13   | 43   DMD_HS1_CLK_N   C13
A13   | 44   DMD_HS1_CLK_P   A13
D10   | 45   DMD_HS1_WDATA0_N   D10
B10   | 46   DMD_HS1_WDATA0_P   B10
C11   | 47   DMD_HS1_WDATA1_N   C11
A11   | 48   DMD_HS1_WDATA1_P   A11
E11   | 49   DMD_HS1_WDATA2_N   E11
F10   | 50   DMD_HS1_WDATA2_P   F10
D12   | 51   DMD_HS1_WDATA3_N   D12
B12   | 52   DMD_HS1_WDATA3_P   B12
D14   | 53   DMD_HS1_WDATA4_N   D14
B14   | 54   DMD_HS1_WDATA4_P   B14
E13   | 55   DMD_HS1_WDATA5_N   E13
F12   | 56   DMD_HS1_WDATA5_P   F12
C15   | 57   DMD_HS1_WDATA6_N   C15
A15   | 58   DMD_HS1_WDATA6_P   A15
E15   | 59   DMD_HS1_WDATA7_N   E15
F14   | 60   DMD_HS1_WDATA7_P   F14
C19   | 61   DMD_HS2_CLK_N   C19
A19   | 62   DMD_HS2_CLK_P   A19
C17   | 63   DMD_HS2_WDATA0_N   C17
A17   | 64   DMD_HS2_WDATA0_P   A17
E17   | 65   DMD_HS2_WDATA1_N   E17
F16   | 66   DMD_HS2_WDATA1_P   F16
D18   | 67   DMD_HS2_WDATA2_N   D18
B18   | 68   DMD_HS2_WDATA2_P   B18
E19   | 69   DMD_HS2_WDATA3_N   E19
F18   | 70   DMD_HS2_WDATA3_P   F18
D20   | 71   DMD_HS2_WDATA4_N   D20
B20   | 72   DMD_HS2_WDATA4_P   B20
C21   | 73   DMD_HS2_WDATA5_N   C21
A21   | 74   DMD_HS2_WDATA5_P   A21
E21   | 75   DMD_HS2_WDATA6_N   E21
F20   | 76   DMD_HS2_WDATA6_P   F20
D22   | 77   DMD_HS2_WDATA7_N   D22
B22   | 78   DMD_HS2_WDATA7_P   B22
J25   | 79   DMD_HS3_CLK_N   J25
H24   | 80   DMD_HS3_CLK_P   H24
C25   | 81   DMD_HS3_WDATA0_N   C25
B24   | 82   DMD_HS3_WDATA0_P   B24
E25   | 83   DMD_HS3_WDATA1_N   E25
D24   | 84   DMD_HS3_WDATA1_P   D24
E23   | 85   DMD_HS3_WDATA2_N   E23
F22   | 86   DMD_HS3_WDATA2_P   F22
G25   | 87   DMD_HS3_WDATA3_N   G25
F24   | 88   DMD_HS3_WDATA3_P   F24
G23   | 89   DMD_HS3_WDATA4_N   G23
H22   | 90   DMD_HS3_WDATA4_P   H22
L25   | 91   DMD_HS3_WDATA5_N   L25
K24   | 92   DMD_HS3_WDATA5_P   K24
J23   | 93   DMD_HS3_WDATA6_N   J23
K22   | 94   DMD_HS3_WDATA6_P   K22
L23   | 95   DMD_HS3_WDATA7_N   L23
M22   | 96   DMD_HS3_WDATA7_P   M22
E1   | 97   DMD_LS0_CLK_N   E1
F2   | 98   DMD_LS0_CLK_P   F2
H4   | 99   DMD_LS0_RDATA   H4
C1   | 100   DMD_LS0_WDATA_N   C1
B2   | 101   DMD_LS0_WDATA_P   B2
G1   | 102   DMD_LS1_CLK   G1
J3   | 103   DMD_LS1_RDATA   J3
E3   | 104   DMD_LS1_WDATA   E3
H2   | 105   DMD_LS2_CLK   H2
M4   | 106   DMD_LS2_RDATA   M4
G3   | 107   DMD_LS2_WDATA   G3
K4   | 108   DMD_LS3_RDATA   K4
U25   | 109   ETM_TRACECLK   U25
T24   | 110   ETM_TRACECTL   T24
AG25   | 111   FLSH_CLK   AG25
AG23   | 112   FLSH_CSZ   AG23
AH22   | 113   FLSH_DATA0   AH22
AH24   | 114   FLSH_DATA1   AH24
AJ25   | 115   FLSH_DATA2   AJ25
AJ23   | 116   FLSH_DATA3   AJ23
AR25   | 117   GPIO_00   AR25
AU25   | 118   GPIO_01   AU25
AW25   | 119   GPIO_02   AW25
AT24   | 120   GPIO_03   AT24
AV24   | 121   GPIO_04   AV24
AR23   | 122   GPIO_05   AR23
AP22   | 123   GPIO_06   AP22
AL23   | 124   GPIO_07   AL23
AM24   | 125   GPIO_08   AM24
P2   | 126   GPIO_09   P2
N3   | 127   GPIO_10   N3
T4   | 128   GPIO_11   T4
V4   | 129   GPIO_12   V4
AD24   | 130   GPIO_13   AD24
AC23   | 131   GPIO_14   AC23
AE25   | 132   GPIO_15   AE25
AE23   | 133   GPIO_16   AE23
AF24   | 134   GPIO_17   AF24
AF22   | 135   GPIO_18   AF22
R1   | 136   GPIO_19   R1
R3   | 137   GPIO_20   R3
U1   | 138   GPIO_21   U1
T2   | 139   GPIO_22   T2
U3   | 140   GPIO_23   U3
W1   | 141   GPIO_24   W1
V2   | 142   GPIO_25   V2
W3   | 143   GPIO_26   W3
AA1   | 144   GPIO_27   AA1
Y4   | 145   GPIO_28   Y4
Y2   | 146   GPIO_29   Y2
AA3   | 147   GPIO_30   AA3
AB4   | 148   GPIO_31   AB4
AC1   | 149   GPIO_32   AC1
AB2   | 150   GPIO_33   AB2
AC3   | 151   GPIO_34   AC3
AD4   | 152   GPIO_35   AD4
AE1   | 153   GPIO_36   AE1
AD2   | 154   GPIO_37   AD2
AE3   | 155   GPIO_38   AE3
AG1   | 156   GPIO_39   AG1
AF4   | 157   GPIO_40   AF4
AF2   | 158   GPIO_41   AF2
AJ1   | 159   GPIO_42   AJ1
AG3   | 160   GPIO_43   AG3
AH2   | 161   GPIO_44   AH2
AJ3   | 162   GPIO_45   AJ3
AL1   | 163   GPIO_46   AL1
AK4   | 164   GPIO_47   AK4
AK2   | 165   GPIO_48   AK2
AN1   | 166   GPIO_49   AN1
AL3   | 167   GPIO_50   AL3
AM2   | 168   GPIO_51   AM2
AA23   | 169   GPTP0   AA23
AB22   | 170   GPTP1   AB22
AC25   | 171   GPTP2   AC25
AK22   | 172   HOST_IRQ   AK22
Y22   | 173   HWTEST_EN   Y22
L3   | 174   IFORCE   L3
AL25   | 175   IIC0_SCL   AL25
AK24   | 176   IIC0_SDA   AK24
V24   | 177   JTAGTCK   V24
Y24   | 178   JTAGTDI   Y24
V22   | 179   JTAGTDO1   V22
W23   | 180   JTAGTDO2   W23
U23   | 181   JTAGTMS1   U23
W25   | 182   JTAGTMS2   W25
AA25   | 183   JTAGTRSTZ   AA25
AB24   | 184   OCLKA   AB24
AN3   | 185   P1_HTPDN   AN3
AM4   | 186   P1_LOCKN   AM4
AU11   | 187   P1_RREF   AU11
AU9   | 188   P1_VX1_D0_N   AU9
AV8   | 189   P1_VX1_D0_P   AV8
AY8   | 190   P1_VX1_D1_N   AY8
BB8   | 191   P1_VX1_D1_P   BB8
AW9   | 192   P1_VX1_D2_N   AW9
BA9   | 193   P1_VX1_D2_P   BA9
AY10   | 194   P1_VX1_D3_N   AY10
BB10   | 195   P1_VX1_D3_P   BB10
AW11   | 196   P1_VX1_D4_N   AW11
BA11   | 197   P1_VX1_D4_P   BA11
AU13   | 198   P1_VX1_D5_N   AU13
AV12   | 199   P1_VX1_D5_P   AV12
AY12   | 200   P1_VX1_D6_N   AY12
BB12   | 201   P1_VX1_D6_P   BB12
AW13   | 202   P1_VX1_D7_N   AW13
BA13   | 203   P1_VX1_D7_P   BA13
AW17   | 204   P2A_LVDS_C_N   AW17
BA17   | 205   P2A_LVDS_C_P   BA17
AW15   | 206   P2A_LVDS_D0_N   AW15
BA15   | 207   P2A_LVDS_D0_P   BA15
AY16   | 208   P2A_LVDS_D1_N   AY16
BB16   | 209   P2A_LVDS_D1_P   BB16
AU15   | 210   P2A_LVDS_D2_N   AU15
AV16   | 211   P2A_LVDS_D2_P   AV16
AY18   | 212   P2A_LVDS_D3_N   AY18
BB18   | 213   P2A_LVDS_D3_P   BB18
AU17   | 214   P2A_LVDS_D4_N   AU17
AV18   | 215   P2A_LVDS_D4_P   AV18
AT16   | 216   P2A_LVDS_RPI   AT16
AW21   | 217   P2B_LVDS_C_N   AW21
BA21   | 218   P2B_LVDS_C_P   BA21
AY20   | 219   P2B_LVDS_D0_N   AY20
BB20   | 220   P2B_LVDS_D0_P   BB20
AU19   | 221   P2B_LVDS_D1_N   AU19
AV20   | 222   P2B_LVDS_D1_P   AV20
AU21   | 223   P2B_LVDS_D2_N   AU21
AV22   | 224   P2B_LVDS_D2_P   AV22
AY22   | 225   P2B_LVDS_D3_N   AY22
BB22   | 226   P2B_LVDS_D3_P   BB22
AW23   | 227   P2B_LVDS_D4_N   AW23
BA23   | 228   P2B_LVDS_D4_P   BA23
AT20   | 229   P2B_LVDS_RPI   AT20
AY6   | 230   P3_DSI_C_N   AY6
BB6   | 231   P3_DSI_C_P   BB6
AW5   | 232   P3_DSI_D0_N   AW5
BA5   | 233   P3_DSI_D0_P   BA5
AY4   | 234   P3_DSI_D1_N   AY4
BB4   | 235   P3_DSI_D1_P   BB4
AU5   | 236   P3_DSI_D2_N   AU5
AV4   | 237   P3_DSI_D2_P   AV4
AW3   | 238   P3_DSI_D3_N   AW3
BA3   | 239   P3_DSI_D3_P   BA3
AV6   | 240   P3_DSI_RCALIB   AV6
AR1   | 241   PARKZ   AR1
N1   | 242   PLL_REFCLK_I   N1
L1   | 243   PLL_REFCLK_O   L1
AP2   | 244   PROJ_ON   AP2
P4   | 245   RESETZ   P4
AN25   | 246   SSP0_CLK   AN25
AM22   | 247   SSP0_CSZ_0   AM22
AN23   | 248   SSP0_DI   AN23
AP24   | 249   SSP0_DO   AP24
T22   | 250   TSTPT_0   T22
R25   | 251   TSTPT_1   R25
R23   | 252   TSTPT_2   R23
P24   | 253   TSTPT_3   P24
N25   | 254   TSTPT_4   N25
P22   | 255   TSTPT_5   P22
N23   | 256   TSTPT_6   N23
M24   | 257   TSTPT_7   M24
AW1   | 258   USB_DAT_N   AW1
AU1   | 259   USB_DAT_P   AU1
AT2   | 260   USB_ID   AT2
AR3   | 261   USB_TXRTUNE   AR3
AP4   | 262   USB_VBUS   AP4
AN15   | 263   VDDA18_FPD   AN15
   |AP16
   |AP18
   |AR19
AM16   | 264   VDDA_CORE_FPD   AM16
   |AM18
   |AM20
K2   | 265   VSENSE   K2
[Model Data]
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[End Model Data]
[End Package Model]
| Models and submodels in the file (72): lvcmos0_nom_1p8_v (I/O), lvcmos1_nom_1p8_h (I/O), lvcmos0_nom_3p3_v (I/O), lvcmos1_nom_3p3_h (I/O), sdio1_r33_1p8_h (I/O), sdio1_r33_3p3_h (I/O), sdio1_r40_1p8_h (I/O), sdio1_r40_3p3_h (I/O), sdio1_r50_1p8_h (I/O), sdio1_r50_3p3_h (I/O), sdio1_r66_1p8_h (I/O), sdio1_r66_3p3_h (I/O), sdio1_utr33_1p8_h (I/O), sdio1_utr33_3p3_h (I/O), sdio1_utr40_1p8_h (I/O), sdio1_utr40_3p3_h (I/O), sdio1_utr50_1p8_h (I/O), sdio1_utr50_3p3_h (I/O), sdio1_utr66_1p8_h (I/O), sdio1_utr66_3p3_h (I/O), IIC33_1_0_V (I/O_open_drain), IIC33_1_1_V (I/O_open_drain), IIC33_1_2_V (I/O_open_drain), IIC33_1_3_V (I/O_open_drain), IIC18_1_0_V (I/O_open_drain), IIC18_1_1_V (I/O_open_drain), IIC18_1_2_V (I/O_open_drain), IIC18_1_3_V (I/O_open_drain), Cell18_0_0_H (I/O_open_drain), Cell18_0_1_H (I/O_open_drain), Cell18_0_2_H (I/O_open_drain), Cell18_0_3_H (I/O_open_drain), Cell33_0_0_H (I/O_open_drain), Cell33_0_1_H (I/O_open_drain), Cell33_0_2_H (I/O_open_drain), Cell33_0_3_H (I/O_open_drain), reset18_0_0 (Input), Cell1_20 (I/O), Cell1_21 (I/O), lvds_tx_01 (Output), lvds_tx_02 (Output), lvds_tx_03 (Output), lvds_tx_04 (Output), lvds_tx_05 (Output), lvds_tx_06 (Output), lvds_tx_07 (Output), lvds_tx_08 (Output), lvds_tx_09 (Output), lvds_tx_10 (Output), lvds_tx_11 (Output), lvds_tx_12 (Output), lvds_tx_13 (Output), lvds_tx_14 (Output), lvds_tx_15 (Output), lvds_tx_16 (Output), lvds_tx_17 (Output), lvds_tx_18 (Output), lvds_tx_19 (Output), lvds_tx_20 (Output), lvds_tx_21 (Output), lvds_tx_22 (Output), lvds_tx_23 (Output), lvds_tx_24 (Output), lvds_rx_01 (Input), lvds_rx_02 (Input), lvcmos_tristate (3-state), lvcmos_tx (Output), lvcmos_rx (Input), FPD_RX_P (Input), FPD_RX_N (Input), VBO_RX_P (Input), VBO_RX_N (Input)
